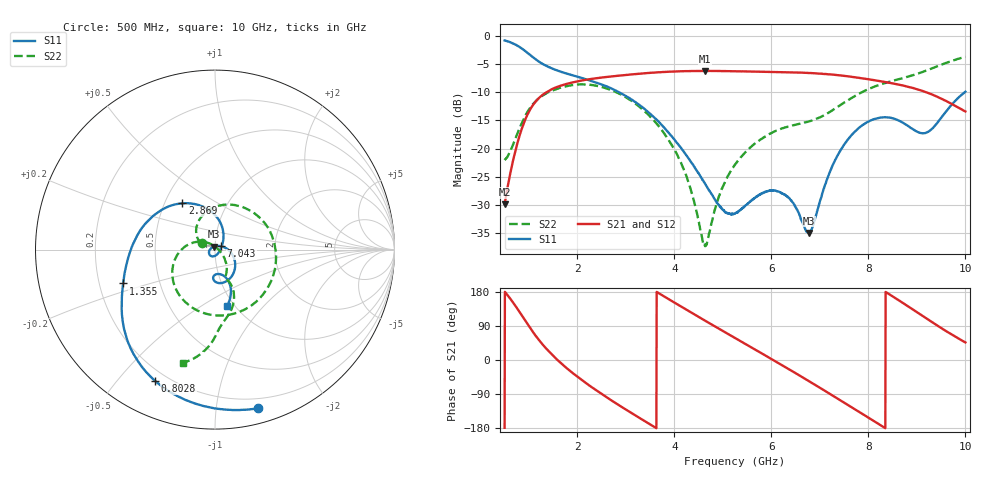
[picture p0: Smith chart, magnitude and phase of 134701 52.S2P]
!  2-Port S-parameters saved by WinCal
! VAR MeasName=S-Parameters (CALIBRATED_DATA) read from VNA (N5242A)
! VAR MeasDate=2013-7-3 16:39:45
! VAR NAME=134701 52
! VAR FILENAME=134701 52.S2P
! VAR DATE=2013-7-3 16:39:45
! VAR PHYS_PORTS=1,2
# Hz S MA R 50
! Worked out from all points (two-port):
!   1601 points, 500 MHz to 10 GHz, reference 50 ohm
!   highest |S21| = -6.18 dB at 4.627 GHz (marker M1); lowest = -29.9 dB at 500 MHz (marker M2)
!   |S21| within 3 dB of the highest: 1.541 GHz to 8.901 GHz (7.36 GHz wide, 141 % of centre)
!   lowest |S11| = -35.0 dB at 6.776 GHz (marker M3), VSWR 1.04, Z = 49.4 + j1.66 ohm
!   |S11| at or under -10 dB: 2.863 GHz to 9.984 GHz (7.121 GHz wide, 111 % of centre)
!   |S22| runs from -37.4 to -3.7 dB; largest |S21 - S12| = 0.002
!   S11 on the Smith chart (normalised r, x): 500 MHz: 0.12, -1.30; 802.8 MHz: 0.15, -0.63; 1.355 GHz: 0.30, -0.16; 2.869 GHz: 0.62, +0.35; 7.043 GHz: 1.07, +0.04; 10 GHz: 0.93, -0.65
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5e8  0.9161 -74.8  0.03183 -178.9  0.03175 -179.1  0.0789 153.5
8.028125e8  0.8042 -114.4  0.1278 127.7  0.1278 127.6  0.1497 134.7
1.105625e9  0.6384 -144.1  0.2509 70.0  0.2506 70.0  0.2548 78.6
1.355e9  0.5451 -159.8  0.3147 30.6  0.3149 30.5  0.3092 32.7
1.681562e9  0.4791 -176.7  0.3652 -10.7  0.3651 -10.8  0.3505 -17.1
2.085312e9  0.4253 163.8  0.4029 -52.2  0.4025 -52.4  0.3728 -65.9
2.47125e9  0.3754 145.2  0.4269 -87.1  0.4257 -87.2  0.3556 -103.5
2.869062e9  0.3152 125.1  0.446 -120.3  0.4447 -120.3  0.3071 -135.9
3.670625e9  0.1739 84.6  0.4774 176.9  0.4764 177.0  0.1592 171.6
4.222812e9  0.09001 58.0  0.4883 134.7  0.4881 134.7  0.06071 139.2
4.626562e9  0.04928 34.6  0.4908 104.3  0.4902 104.3  0.01374 52.7
4.947188e9  0.03002 2.4  0.4897 80.4  0.4899 80.4  0.04038 -27.3
5.25e9  0.02631 -45.3  0.4872 58.0  0.4875 58.0  0.07192 -42.6
6.099062e9  0.04193 -133.5  0.4802 -4.6  0.4801 -4.6  0.1438 -63.7
6.41375e9  0.03431 -163.3  0.4773 -28.2  0.4776 -28.3  0.1592 -68.4
6.775938e9  0.01771 109.0  0.4701 -55.9  0.4701 -55.9  0.1744 -68.9
6.835312e9  0.01942 85.0  0.4693 -60.6  0.4691 -60.5  0.1774 -68.5
7.043125e9  0.03914 28.5  0.4631 -76.7  0.4631 -76.7  0.1934 -66.7
7.642812e9  0.1303 -31.2  0.4351 -123.9  0.4355 -123.9  0.2797 -67.8
8.420625e9  0.1889 -81.4  0.3858 174.3  0.3854 174.1  0.3914 -81.4
9.1925e9  0.1385 -80.0  0.317 110.1  0.3166 109.9  0.4947 -90.5
1e10  0.3203 -77.8  0.2138 46.4  0.2139 46.1  0.6551 -105.7
